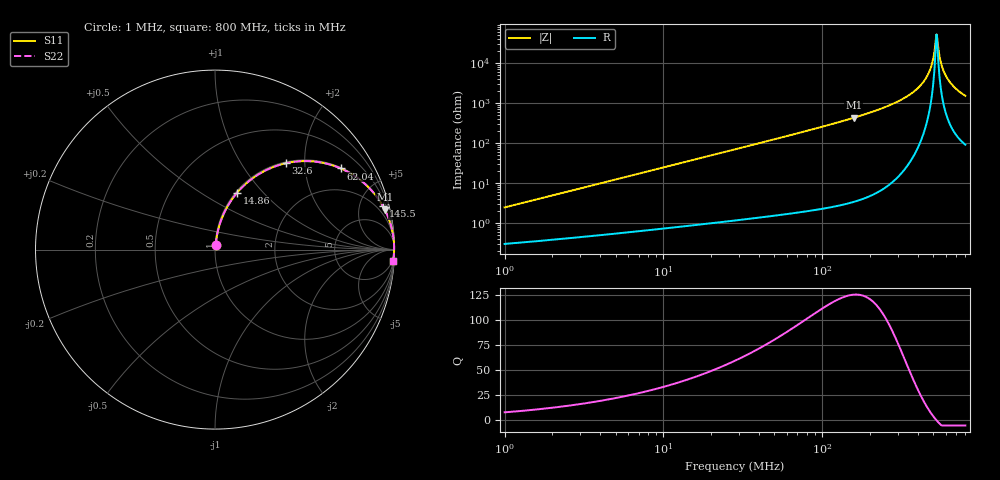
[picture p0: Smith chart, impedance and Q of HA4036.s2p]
# MHz S MA R 50
!Freq  MagS11  AngS11  MagS21  AngS21  MagS12  AngS12  MagS22  AngS22
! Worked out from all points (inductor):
!   801 points, 1 MHz to 800 MHz, reference 50 ohm
!   read as one part in series: L = 390 nH near 1.034 MHz
!   highest Q = 126 at 158.2 MHz (marker M1), where L = 429 nH
!   self-resonance near 526.8 MHz
!   S11 on the Smith chart (normalised r, x): 1 MHz: 1.01, +0.05; 14.86 MHz: 1.02, +0.73; 32.6 MHz: 1.02, +1.60; 62.04 MHz: 1.03, +3.08; 145.5 MHz: 1.06, +7.72; 800 MHz: 3, -30
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1  0.02461 81.6  0.9967 -1.4  0.9967 -1.4  0.02461 81.6
3.063851  0.07467 82.3  0.9927 -4.3  0.9927 -4.3  0.07467 82.3
9.30907  0.2211 75.5  0.9684 -12.8  0.9684 -12.8  0.2211 75.5
14.86355  0.34 68.8  0.9324 -19.9  0.9324 -19.9  0.34 68.8
28.28427  0.5664 54.5  0.8147 -34.5  0.8147 -34.5  0.5664 54.5
32.60136  0.621 50.7  0.7742 -38.4  0.7742 -38.4  0.621 50.7
62.03804  0.8347 32.8  0.5414 -56.6  0.5414 -56.6  0.8347 32.8
86.65878  0.9059 24.5  0.415 -64.9  0.415 -64.9  0.9059 24.5
145.4796  0.9662 14.5  0.2503 -75.0  0.2503 -75.0  0.9662 14.5
158.1578  0.9718 13.2  0.2282 -76.4  0.2282 -76.4  0.9718 13.2
263.3003  0.9921 6.6  0.1154 -82.8  0.1154 -82.8  0.9921 6.6
355.7053  0.9968 3.6  0.06225 -85.3  0.06225 -85.3  0.9968 3.6
431.0763  0.998 1.8  0.03128 -85.5  0.03128 -85.5  0.998 1.8
480.5398  0.9982 0.8  0.01437 -82.4  0.01437 -82.4  0.9982 0.8
496.8723  0.9982 0.5  0.009265 -78.4  0.009265 -78.4  0.9982 0.5
513.76  0.9981 0.2  0.004347 -64.2  0.004347 -64.2  0.9981 0.2
526.8013  0.9981 0.0  0.001948 -1.4  0.001948 -1.4  0.9981 0.0
540.1737  0.998 -0.2  0.004328 61.9  0.004328 61.9  0.998 -0.2
572.711  0.9977 -0.7  0.01306 79.5  0.01306 79.5  0.9977 -0.7
607.2081  0.9973 -1.3  0.02209 82.4  0.02209 82.4  0.9973 -1.3
682.5612  0.9962 -2.3  0.04044 83.4  0.04044 83.4  0.9962 -2.3
800  0.9938 -3.8  0.06619 82.8  0.06619 82.8  0.9938 -3.8
